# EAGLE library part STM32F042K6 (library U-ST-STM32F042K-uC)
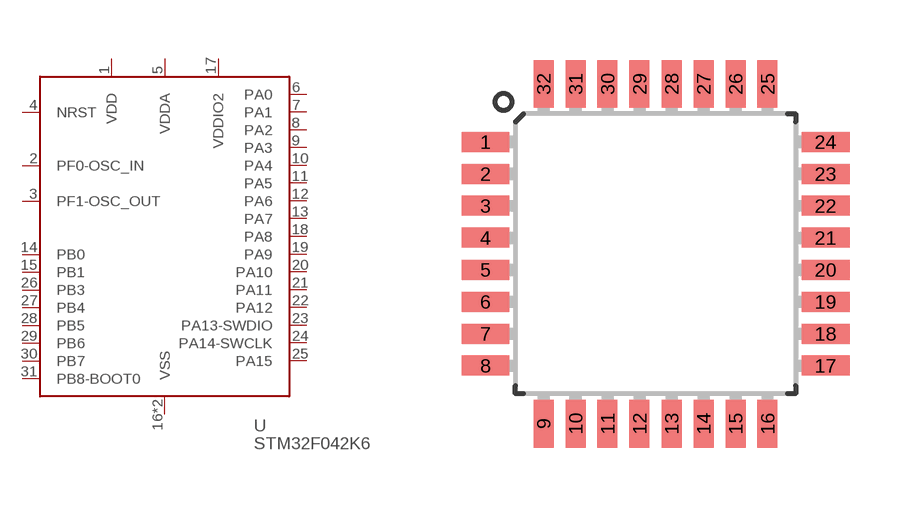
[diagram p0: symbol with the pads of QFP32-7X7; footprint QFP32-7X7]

Designator prefix U

## STM32F042K6  [QFP32-7X7]
1  VDD  pwr
2  PF0-OSC_IN
3  PF1-OSC_OUT
4  NRST
5  VDDA  pwr
6  PA0
7  PA1
8  PA2
9  PA3
10  PA4
11  PA5
12  PA6
13  PA7
14  PB0
15  PB1
16  VSS  pwr
17  VDDIO2  pwr
18  PA8
19  PA9
20  PA10
21  PA11
22  PA12
23  PA13-SWDIO
24  PA14-SWCLK
25  PA15
26  PB3
27  PB4
28  PB5
29  PB6
30  PB7
31  PB8-BOOT0
32  VSS  pwr

## Footprint QFP32-7X7 (pad centres in mm)
smd 1.2 x 0.5: 1 -4.25,2.8; 2 -4.25,2; 3 -4.25,1.2; 4 -4.25,0.4; 5 -4.25,-0.4; 6 -4.25,-1.2; 7 -4.25,-2; 8 -4.25,-2.8; 17 4.25,-2.8; 18 4.25,-2; 19 4.25,-1.2; 20 4.25,-0.4; 21 4.25,0.4; 22 4.25,1.2; 23 4.25,2; 24 4.25,2.8
smd 0.5 x 1.2: 9 -2.8,-4.25; 10 -2,-4.25; 11 -1.2,-4.25; 12 -0.4,-4.25; 13 0.4,-4.25; 14 1.2,-4.25; 15 2,-4.25; 16 2.8,-4.25; 25 2.8,4.25; 26 2,4.25; 27 1.2,4.25; 28 0.4,4.25; 29 -0.4,4.25; 30 -1.2,4.25; 31 -2,4.25; 32 -2.8,4.25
